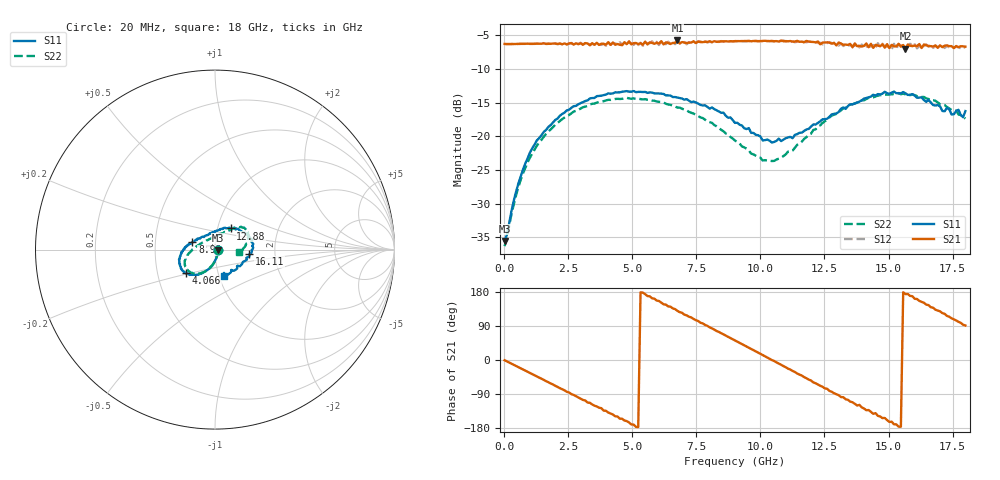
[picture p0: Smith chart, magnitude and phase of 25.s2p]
!Agilent Technologies,N5230A,US43500223,A.07.50.48
!Agilent N5230A: A.07.50.48
!Date: Thursday, January 14, 2016 11:59:46
!Correction: S11(Full 2 Port(1,2))
!S21(Full 2 Port(1,2))
!S12(Full 2 Port(1,2))
!S22(Full 2 Port(1,2))
!S2P File: Measurements: S11, S21, S12, S22:
# Hz S  dB  R 50
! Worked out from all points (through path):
!   201 points, 20 MHz to 18 GHz, reference 50 ohm
!   highest |S21| = -5.74 dB at 6.763 GHz (marker M1); lowest = -7.0 dB at 15.66 GHz (marker M2)
!   group delay of S21, straight-line fit = 97.1 ps
!   lowest |S11| = -35.5 dB at 20 MHz (marker M3), VSWR 1.03, Z = 51.7 - j0.187 ohm
!   |S11| at or under -10 dB: start of sweep to end of sweep
!   |S22| runs from -36.3 to -13.6 dB; largest |S21 - S12| = 0.055
!   S11 on the Smith chart (normalised r, x): 20 MHz: 1.03, -0.00; 4.066 GHz: 0.70, -0.19; 8.92 GHz: 0.77, +0.06; 12.88 GHz: 1.16, +0.28; 16.11 GHz: 1.47, -0.07; 18 GHz: 1.06, -0.32
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2e7  -35.55 -6.2  -6.26 -0.6  -6.28 -0.9  -36.31 -0.9
5.594e8  -26.98 -79.2  -6.25 -18.8  -6.26 -19.0  -27.52 -77.3
1.0988e9  -21.76 -96.9  -6.25 -37.2  -6.25 -37.4  -22.54 -95.2
1.9978e9  -17.55 -113.6  -6.19 -68.1  -6.17 -69.0  -18.27 -111.2
3.0766e9  -14.92 -129.0  -6.38 -105.4  -6.31 -105.8  -15.67 -125.3
4.0655e9  -13.60 -140.6  -5.98 -138.6  -6.09 -138.0  -14.56 -137.0
5.1443e9  -13.42 -152.8  -6.12 -176.5  -6.05 -177.7  -14.42 -149.8
6.0433e9  -13.62 -162.7  -6.21 155.7  -6.43 153.2  -14.86 -159.0
6.7625e9  -14.22 -170.9  -5.74 129.6  -5.82 129.3  -15.71 -165.6
7.8413e9  -15.38 176.6  -5.95 92.6  -5.85 91.0  -17.52 -177.0
8.9201e9  -17.57 162.2  -5.88 54.8  -5.87 53.1  -20.31 165.1
9.01e9  -17.99 159.6  -5.83 51.6  -5.87 50.1  -20.62 163.4
1.04484e10  -20.91 115.6  -5.82 -0.1  -5.84 -1.9  -23.66 111.3
1.11676e10  -20.07 94.7  -5.82 -25.2  -5.90 -28.0  -22.28 82.3
1.20666e10  -18.22 71.4  -5.96 -59.1  -5.95 -59.9  -19.05 61.6
1.28757e10  -16.65 53.4  -6.09 -87.8  -6.22 -89.4  -16.77 50.7
1.39545e10  -14.63 31.2  -6.65 -124.9  -6.35 -125.6  -14.63 42.3
1.50333e10  -13.67 12.1  -6.87 -163.4  -6.68 -165.7  -13.76 34.2
1.56626e10  -13.59 0.3  -6.97 173.9  -6.55 173.2  -13.76 27.1
1.61121e10  -14.26 -7.2  -6.58 161.0  -6.90 156.1  -14.02 21.7
1.7101e10  -16.22 -35.5  -6.73 123.8  -6.51 120.1  -15.24 7.6
1.8e10  -16.23 -70.6  -6.66 91.0  -6.85 86.7  -17.36 -6.5
